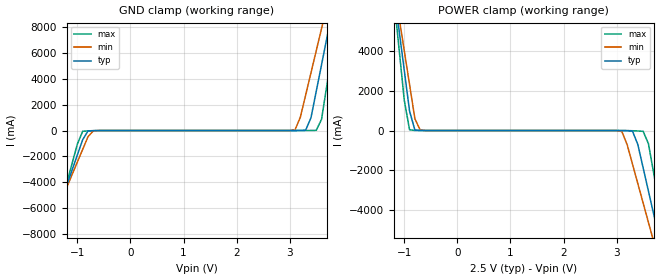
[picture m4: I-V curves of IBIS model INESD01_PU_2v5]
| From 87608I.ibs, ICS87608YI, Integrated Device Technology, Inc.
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[Model] INESD01_PU_2v5
Model_type   Input
Polarity   Non-Inverting
Vinl = 1.4V
Vinh = 1.85V
|   typ   min   max
C_comp   2pF   1.5pF   2.5pF
|   typ   min   max
[Voltage range]  2.5V   2.375V   2.625V
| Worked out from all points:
|   GND clamp passes 1 mA (typ) near -0.54 V on its own axis
|   POWER clamp passes 1 mA (typ) near -0.66 V on its own axis
[GND_clamp]
|Voltage   I(typ)   I(min)   I(max)
-2.5V     -19.6A     -17.18A    -23.67A
-1.6V     -8.969A    -8.332A    -10.1A
-1.5V     -7.788A    -7.349A    -8.588A
-900mV    -707.1mA   -1.46A     -57.43mA
-700mV    -7.027mA   -24.05mA   -13.28mA
3.1V      199.2uA    53.94mA    11.78uA
3.3V      28.4mA     2.748A     652.4uA
3.5V      3.045A     6.192A     15.72mA
3.6V      5.115A     7.914A     872.4mA
3.7V      7.185A     9.638A     3.52A
3.9V      11.33A     13.09A     8.818A
5V        34.14A     32.07A     37.99A
[POWER_clamp]
|Voltage   I(typ)   I(min)   I(max)
-1.5V     9.257A     9.207A     9.48A
-1.2V     7.185A     7.484A     6.83A
-1.1V     5.115A     5.761A     4.182A
-900mV    976.9mA    2.318A     34.23mA
-700mV    1.582mA    24.31mA    1.044mA
3.1V      -2.107mA   -51.03mA   -534.5uA
3.3V      -35.62mA   -1.705A    -10.86mA
3.5V      -1.886A    -3.666A    -39.41mA
3.6V      -3.066A    -4.647A    -666.9mA
3.8V      -5.426A    -6.612A    -3.684A
3.9V      -6.607A    -7.595A    -5.193A
5V        -19.6A     -18.41A    -21.79A
